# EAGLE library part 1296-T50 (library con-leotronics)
1.27mm SINGLE ROW FEMALE SOCKET Source: http://www.leotronics.co.uk/Conexcon/Data%20Sheets/sec.%20A/1296ing.pdf
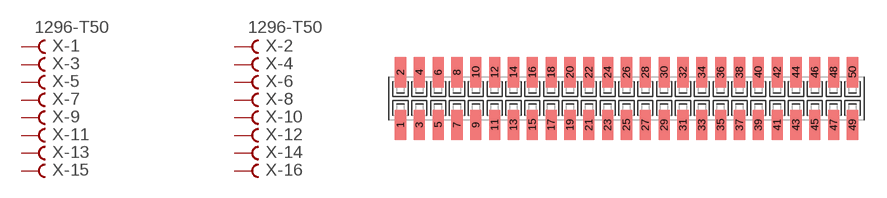
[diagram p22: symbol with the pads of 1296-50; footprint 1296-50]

Designator prefix X; gates -1=FVAL -2=FVAL -3=F -4=F -5=F -6=F -7=F -8=F -9=F -10=F -11=F -12=F -13=F -14=F -15=F -16=F -17=F -18=F -19=F -20=F -21=F -22=F -23=F -24=F -25=F -26=F -27=F -28=F -29=F -30=F -31=F -32=F -33=F -34=F -35=F -36=F -37=F -38=F -39=F -40=F -41=F -42=F -43=F -44=F -45=F -46=F -47=F -48=F -49=F -50=F

## 1296-T50 (OC_FARNELL: unknown; OC_NEWARK: unknown)  [1296-50]
1  -1:B  pas
2  -2:B  pas
3  -3:B  pas
4  -4:B  pas
5  -5:B  pas
6  -6:B  pas
7  -7:B  pas
8  -8:B  pas
9  -9:B  pas
10  -10:B  pas
11  -11:B  pas
12  -12:B  pas
13  -13:B  pas
14  -14:B  pas
15  -15:B  pas
16  -16:B  pas
17  -17:B  pas
18  -18:B  pas
19  -19:B  pas
20  -20:B  pas
21  -21:B  pas
22  -22:B  pas
23  -23:B  pas
24  -24:B  pas
25  -25:B  pas
26  -26:B  pas
27  -27:B  pas
28  -28:B  pas
29  -29:B  pas
30  -30:B  pas
31  -31:B  pas
32  -32:B  pas
33  -33:B  pas
34  -34:B  pas
35  -35:B  pas
36  -36:B  pas
37  -37:B  pas
38  -38:B  pas
39  -39:B  pas
40  -40:B  pas
41  -41:B  pas
42  -42:B  pas
43  -43:B  pas
44  -44:B  pas
45  -45:B  pas
46  -46:B  pas
47  -47:B  pas
48  -48:B  pas
49  -49:B  pas
50  -50:B  pas

## Footprint 1296-50 (pad centres in mm)
1.27mm SINGLE ROW FEMALE SOCKET Source: http://www.leotronics.co.uk/Conexcon/Data%20Sheets/sec.%20A/1296ing.pdf
smd 0.76 x 2.05: 1 -15.24,-1.78; 2 -15.24,1.78; 3 -13.97,-1.78; 4 -13.97,1.78; 5 -12.7,-1.78; 6 -12.7,1.78; 7 -11.43,-1.78; 8 -11.43,1.78; 9 -10.16,-1.78; 10 -10.16,1.78; 11 -8.89,-1.78; 12 -8.89,1.78; 13 -7.62,-1.78; 14 -7.62,1.78; 15 -6.35,-1.78; 16 -6.35,1.78; 17 -5.08,-1.78; 18 -5.08,1.78; 19 -3.81,-1.78; 20 -3.81,1.78; 21 -2.54,-1.78; 22 -2.54,1.78; 23 -1.27,-1.78; 24 -1.27,1.78; 25 0,-1.78; 26 0,1.78; 27 1.27,-1.78; 28 1.27,1.78; 29 2.54,-1.78; 30 2.54,1.78; 31 3.81,-1.78; 32 3.81,1.78; 33 5.08,-1.78; 34 5.08,1.78; 35 6.35,-1.78; 36 6.35,1.78; 37 7.62,-1.78; 38 7.62,1.78; 39 8.89,-1.78; 40 8.89,1.78; 41 10.16,-1.78; 42 10.16,1.78; 43 11.43,-1.78; 44 11.43,1.78; 45 12.7,-1.78; 46 12.7,1.78; 47 13.97,-1.78; 48 13.97,1.78; 49 15.24,-1.78; 50 15.24,1.78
